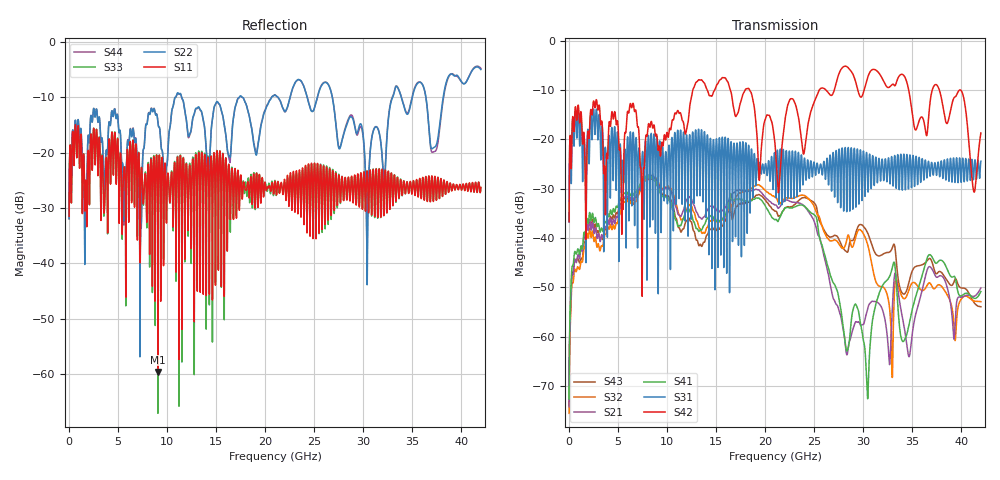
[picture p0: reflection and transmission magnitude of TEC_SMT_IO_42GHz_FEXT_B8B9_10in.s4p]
!! CHANNEL DESCRIPTION: Next Generation 28Gbps High Density SMT I/O Connector
!!  with 10" 5-6-5 Megatron 6 Stripline trace on host side and 1.25" 7-5-7 Megtron 6 Microstrip trace on plug side at 14GHz
!! HOST PCB DESCRIPTION: PCB thickness 2.86 mm, Nelco 4000-13SI (Dk 3.32, Df 0.010)
!!  23 Layer Board, 12 GND planes, 2 Layer route-out on Layers 10,12, 8 mil stub on vias
!!  Pairs on following layers
!!  Layer 10 - B8B9
!! CONNECTOR DESCRIPTION:  Next Generation 28Gbps High Density SMT I/O Connector
!! PLUG-IN CARD DESCRIPTION:  PCB thickness 1mm thick, Nelco 4000-13SI (Dk 3.32, Df 0.010)
!!  6 Layer Board, 4 GND planes, 0.35 x 1.4mm mating pads
!!  Micro-strip diff traces referenced to GND plane 3mils down, 2nd GND plane 15mils from top of board
!!  PCB GND planes are symmetric
!! MODEL DESCRIPTION: TE Connectivity S-parameter model produced from Macro-model
!! MODEL DATE: 9/25/2014 CR1a_GC1i, VR6&12_4
!! MODEL STATUS: Developmental
!! MODEL GEOMETRY: 2 Rows - Rows A, B. 3 pairs in each row, 6 total pairs
!! MODEL FREQUENCY RANGE: DC to 42 GHz in 10 MHz frequency steps
!! MODEL EDGE RATE LIMITATION: 11.90 ps (Using conservative 0.5/Fmax rule of thumb)
!! TIME-DOMAIN TRANSFORM CAUTIONS:
!! 1.) Do not simulate transient edge rates faster than the number listed above.  Edge
!!  rates faster than this number contain significant spectral content at frequencies
!!  above the model's highest frequency.
!! 2.) Even when simulating edge rates that are slower than the number listed above, be
!!  aware that the best time resolution possible with a direct iFFT is (1 / 2Fmax).
!!  As a result, time resolution is typically not adequate for most time-domain
!!  simulations unless tricks such as frequency-domain zero-padding and windowing are
!!  used to minimize leakage and aliasing.
!! 3.) Because the model has a uniform frequency step, a direct iFFT will result in an
!!  impulse that that has a time length given by either (1 / Fstep) or (1 / 2Fstep),
!!  depending on the transform being used.  Care has been taken in selecting the
!!  frequency step to ensure a settled impulse response for the model.  Therefore,
!!  convolution with the model's impulse response should present no issues.  However,
!!  if directly concatenating s-parameter models in the frequency domain a user must
!!  either interpolate necessary interim frequencies or complete impulse response
!!  zero-padding.  Impulse response zero-padding is more difficult, but more accurate.
!! PORT DEFINITIONS:
!! Port  1  ----->  Host, Bot Row  B8  B5  Module, Top Row  <-----  Port  2
!! Port  3  ----->  Host, Bot Row  B9  B6  Module, Top Row  <-----  Port  4
# Hz S MA R 50
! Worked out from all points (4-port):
!   4200 points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, 10 MHz to 42 GHz, reference 50 ohm
!   strongest paths, dB at 10 MHz, 10.51 GHz, 21.01 GHz, 31.51 GHz, 42 GHz:
!     S42: -36.7, -16.2, -21.0, -6.3, -18.7
!     S31: -36.8, -19.7, -24.2, -26.4, -24.4
!     S41: -72.7, -34.0, -36.3, -51.9, -50.9
!     S21: -74.2, -31.3, -33.3, -53.1, -50.1
!     S32: -75.6, -30.7, -31.7, -49.6, -52.9
!     S43: -74.0, -33.4, -34.6, -43.6, -54.0
!   lowest |S11| = -59.6 dB at 9.07 GHz (marker M1), VSWR 1.00, Z = 50 + j0.103 ohm
!   |S11| at or under -10 dB: start of sweep to end of sweep
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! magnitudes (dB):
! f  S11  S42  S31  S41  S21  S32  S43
! 10 MHz  -31.5  -36.7  -36.8  -72.7  -74.2  -75.6  -74.0
! 1.96 GHz  -19.6  -18.4  -18.6  -37.0  -38.5  -40.0  -38.2
! 9.07 GHz  -59.6  -22.0  -29.0  -29.6  -29.0  -28.7  -29.3
! 25.01 GHz  -22.2  -12.4  -24.8  -35.3  -36.7  -33.6  -32.9
! 30.42 GHz  -23.7  -7.7  -25.3  -72.1  -54.7  -41.1  -38.9
! 33.06 GHz  -28.4  -8.8  -29.4  -45.2  -50.9  -58.9  -41.5
! 42 GHz  -26.3  -18.7  -24.4  -50.9  -50.1  -52.9  -54.0
